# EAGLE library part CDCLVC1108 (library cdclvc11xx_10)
CDCLVC1108 3.3V and 2.5V LVCMOS High-Performance Clock Buffer - 1:8 Fan-out Source: http://www.ti.com/lit/ds/symlink/cdclvc1108.pdf
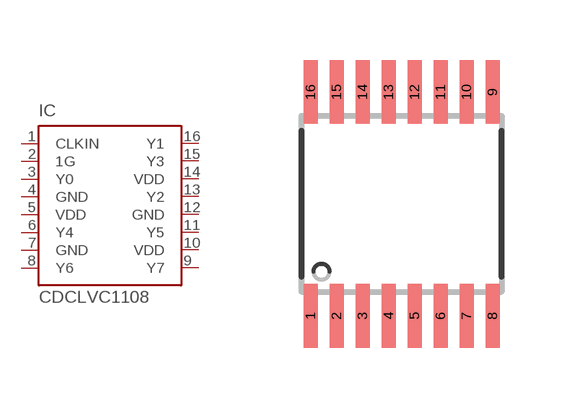
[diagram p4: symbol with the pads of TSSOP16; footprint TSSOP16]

Designator prefix IC

## CDCLVC1108PW (MF: Texas Instruments; MPN: CDCLVC1108; OC_FARNELL: 1829684; OC_NEWARK: 23T0797)  [TSSOP16]
1  CLKIN  in
2  1G  in
3  Y0  out
4  GND  pwr
5  VDD  pwr
6  Y4  out
7  GND  pwr
8  Y6  out
9  Y7  out
10  VDD  pwr
11  Y5  out
12  GND  pwr
13  Y2  out
14  VDD  pwr
15  Y3  out
16  Y1  out

## Footprint TSSOP16 (pad centres in mm)
TSSOP-16 Plastic Thin Srink Small Outline (PW) Source: http://www.ti.com/lit/ds/symlink/cdclvc1108.pdf
smd 0.35 x 1.6: 1 -2.275,-2.8; 2 -1.625,-2.8; 3 -0.975,-2.8; 4 -0.325,-2.8; 5 0.325,-2.8; 6 0.975,-2.8; 7 1.625,-2.8; 8 2.275,-2.8; 9 2.275,2.8; 10 1.625,2.8; 11 0.975,2.8; 12 0.325,2.8; 13 -0.325,2.8; 14 -0.975,2.8; 15 -1.625,2.8; 16 -2.275,2.8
